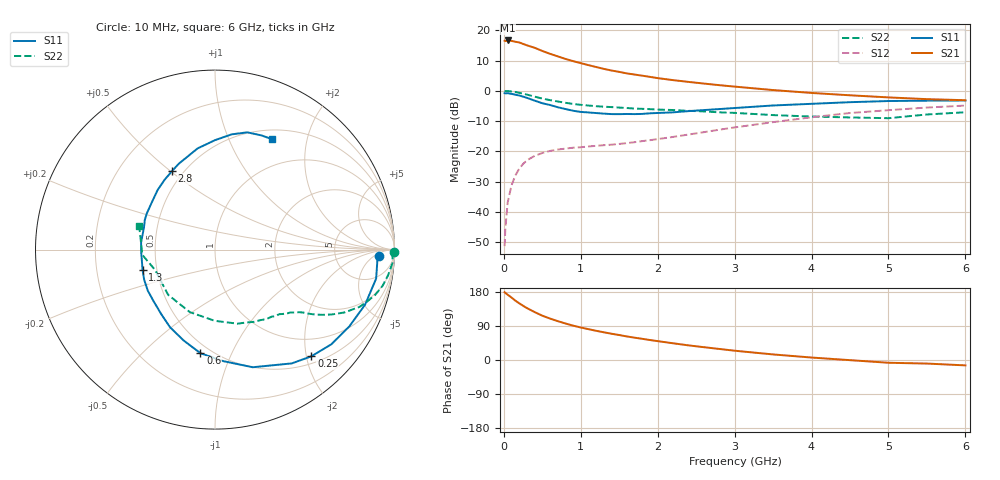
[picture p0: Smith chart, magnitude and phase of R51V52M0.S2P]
! SIEMENS Small Signal Semiconductors
! BFR183
! Si NPN RF Bipolar Junction Transistor in SOT23
! VCE = 1.5 V  IC = 2 mA
! Common Emitter S-Parameters:  May  1996
# GHz  S  MA  R  50
!  f  S11  S21  S12  S22
! GHz  MAG  ANG  MAG  ANG  MAG  ANG  MAG  ANG
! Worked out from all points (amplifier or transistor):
!   36 points, 10 MHz to 6 GHz, reference 50 ohm
!   highest |S21| = 16.7 dB at 50 MHz (marker M1)
!   |S21| within 3 dB of that: start of sweep to 455.4 MHz
!   unconditionally stable (mu >= 1): 1.363 GHz to 2.909 GHz
!   at 250 MHz: K = 0.23, MSG = 19.8 dB, |S12| = -24.2 dB
!   at 1.4 GHz: K = 1.02, MAG = 11.4 dB, |S12| = -17.8 dB
!   at 6 GHz: K = 0.93, MSG = 0.9 dB, |S12| = -4.9 dB
!   S11 on the Smith chart (normalised r, x): 10 MHz: 19, -7; 250 MHz: 0.63, -2.09; 600 MHz: 0.44, -0.77; 1.3 GHz: 0.42, -0.12; 2.8 GHz: 0.44, +0.51; 6 GHz: 0.62, +1.46
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0.01  0.9118 -2.1  6.721 178.9  0.0027 91.0  0.9961 -0.9
0.02  0.9067 -4.0  6.624 176.9  0.0054 87.3  0.99 -1.7
0.05  0.9122 -10.2  6.8 172.3  0.0143 83.6  0.9915 -4.3
0.1  0.8908 -20.1  6.688 164.8  0.0275 78.1  0.9749 -8.4
0.15  0.8623 -29.7  6.469 156.6  0.0399 73.4  0.9554 -12.2
0.2  0.836 -39.1  6.301 149.6  0.0516 68.5  0.9273 -15.8
0.25  0.8012 -47.9  5.963 143.1  0.0618 63.8  0.8945 -19.0
0.3  0.7648 -56.0  5.65 137.0  0.0709 60.4  0.8665 -21.6
0.4  0.6884 -72.2  5.149 126.5  0.084 53.9  0.8017 -25.9
0.5  0.623 -85.8  4.56 116.9  0.0937 49.0  0.7435 -29.1
0.6  0.5829 -98.0  4.089 109.4  0.1014 45.7  0.7016 -31.2
0.8  0.4998 -120.1  3.367 96.4  0.1108 41.4  0.634 -34.3
0.9  0.4687 -129.5  3.098 90.7  0.1145 41.0  0.6063 -35.4
1.1  0.4388 -148.6  2.659 81.4  0.1202 40.9  0.5708 -37.8
1.3  0.4194 -164.0  2.305 73.1  0.1262 41.4  0.546 -39.9
1.7  0.4119 167.8  1.857 58.9  0.1414 45.9  0.5085 -45.0
2.2  0.4406 142.6  1.502 44.1  0.1728 50.3  0.4813 -53.5
2.8  0.4989 118.6  1.24 29.2  0.2275 51.5  0.4408 -67.2
3.5  0.5722 99.7  1.029 14.7  0.3035 47.1  0.3968 -90.2
4.5  0.6486 81.8  0.843 -0.4  0.4294 34.9  0.3628 -136.0
5.5  0.6869 67.8  0.728 -9.4  0.5288 20.6  0.4061 -175.9
6  0.6927 62.5  0.699 -14.2  0.5701 11.5  0.4423 162.7
